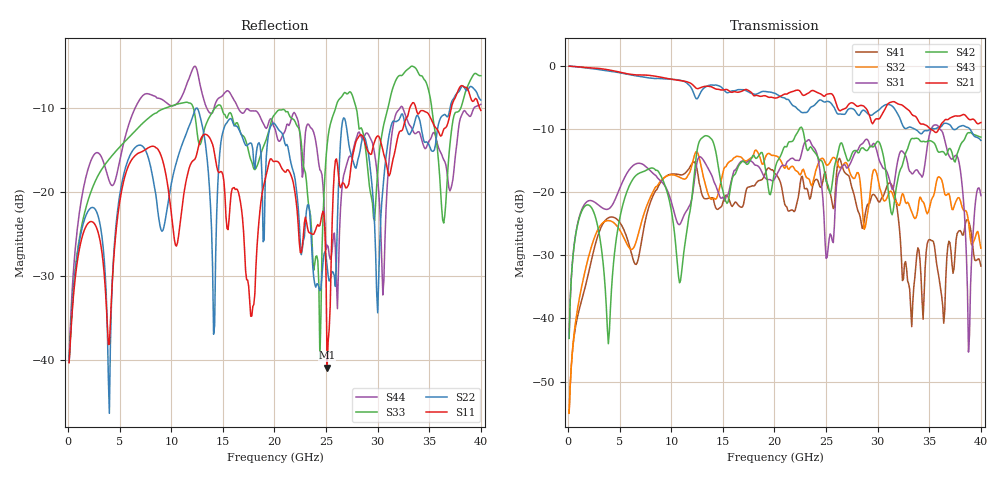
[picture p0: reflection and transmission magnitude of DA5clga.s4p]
! ADC12DJ3200QML-SP
! 196-pin ZMX package
! CLGA Ceramic Package without columns (ceramic land grid array)
! Texas Instruments 4/21/2021
! Single-ended  S-parameters
! PORT#  PORT_NAME  NET_NAME
! PORT1:  DAxN.DIEBUMP DAxN
! PORT2:  DAxN.BGA  DAxN
! PORT3:  DAxP.DIEBUMP DAxP
! PORT4:  DAxP.BGA  DAxP
! Touchstone Ver. 1.0
! Number of ports is 4
# Hz	S	MA	R	50.000000
! SCATTERING PARAMETERS  :
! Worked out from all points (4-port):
!   400 points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, 100 MHz to 40 GHz, reference 50 ohm
!   strongest paths, dB at 100 MHz, 10.1 GHz, 20.1 GHz, 30.1 GHz, 40 GHz:
!     S21: -0.1, -2.2, -5.1, -8.4, -9.0
!     S43: -0.1, -2.2, -4.4, -7.0, -11.8
!     S42: -43.1, -23.9, -16.0, -12.0, -11.3
!     S31: -43.1, -22.1, -17.6, -14.7, -20.6
!     S32: -55.0, -17.3, -14.3, -18.5, -28.9
!     S41: -55.0, -17.1, -17.1, -21.6, -31.7
!   lowest |S11| = -40.9 dB at 25.1 GHz (marker M1), VSWR 1.02, Z = 49.2 - j0.428 ohm
!   |S11| at or under -10 dB: start of sweep to 33.12 GHz; 33.69 GHz to 37.14 GHz (3.449 GHz wide, 9.74 % of centre); 39.87232 GHz to end of sweep
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1e8  0.009619 -25.1  0.9908 -3.7  0.006985 77.6  0.001786 -131.8
     0.9908 -3.7  0.009765 -25.8  0.001776 -131.1  0.006959 76.5
     0.006985 77.6  0.001776 -131.1  0.009843 -31.0  0.9908 -3.8
     0.001786 -131.8  0.006959 76.5  0.9908 -3.8  0.01044 -30.7
4.8e9  0.07087 -65.4  0.8959 -170.9  0.09735 36.9  0.06022 58.3
       0.8959 -170.9  0.07749 -71.8  0.05309 48.4  0.05007 110.2
       0.09735 36.9  0.05309 48.4  0.1789 -33.1  0.8849 -172.5
       0.06022 58.3  0.05007 110.2  0.8849 -172.5  0.1333 -113.7
1.02e10  0.058 50.7  0.7775 4.1  0.07322 -42.7  0.139 -112.0
         0.7775 4.1  0.1275 -111.5  0.1367 -125.8  0.05618 -61.0
         0.07322 -42.7  0.1367 -125.8  0.3266 -16.8  0.7781 1.1
         0.139 -112.0  0.05618 -61.0  0.7781 1.1  0.325 -161.4
2.44e10  0.06304 -81.7  0.6021 -114.6  0.1476 -12.6  0.1104 95.5
         0.6021 -114.6  0.02576 161.2  0.1788 78.9  0.1787 -14.8
         0.1476 -12.6  0.1788 78.9  0.01015 -39.9  0.5362 -113.1
         0.1104 95.5  0.1787 -14.8  0.5362 -113.1  0.135 98.3
2.51e10  0.008996 -151.1  0.5951 -138.2  0.03038 30.9  0.1147 56.9
         0.5951 -138.2  0.03601 88.7  0.1629 43.9  0.1176 -11.8
         0.03038 30.9  0.1629 43.9  0.1896 35.8  0.5219 -141.3
         0.1147 56.9  0.1176 -11.8  0.5219 -141.3  0.04814 112.2
3.88e10  0.3984 -147.4  0.3785 114.5  0.005419 -153.8  0.05894 -50.0
         0.3785 114.5  0.4094 -133.3  0.05846 -99.1  0.2952 -13.3
         0.005419 -153.8  0.05846 -99.1  0.436 -128.9  0.3226 110.7
         0.05894 -50.0  0.2952 -13.3  0.3226 110.7  0.285 -166.9
4e10  0.3045 170.1  0.3548 67.0  0.09379 -0.2  0.02598 -137.5
      0.3548 67.0  0.3511 -152.0  0.03594 -101.2  0.272 -26.8
      0.09379 -0.2  0.03594 -101.2  0.4901 -176.9  0.2561 67.8
      0.02598 -137.5  0.272 -26.8  0.2561 67.8  0.3314 -178.4
